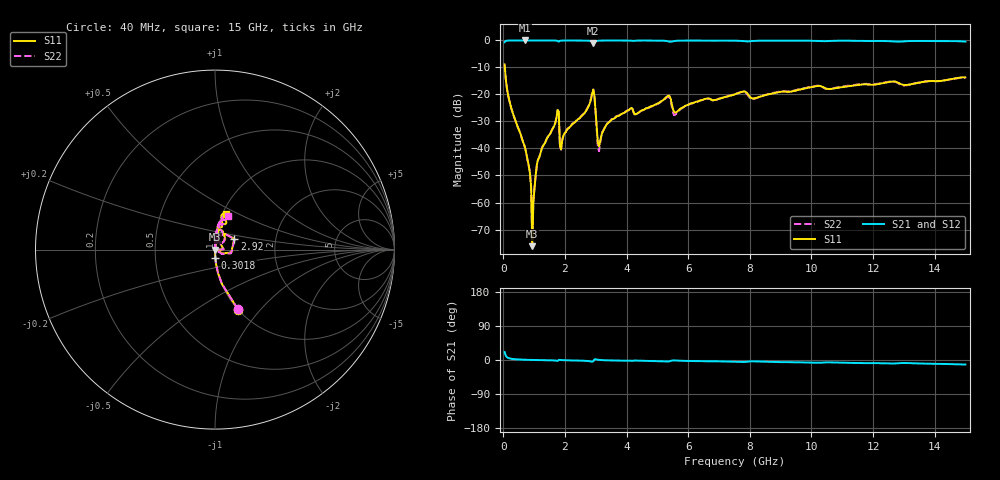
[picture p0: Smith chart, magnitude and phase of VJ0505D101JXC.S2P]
! VJ0505D101JXC
! MLCC placed on 25 mil thick microstrip substrate in series configuraton.
! DATE 06/29/2018  09:30
! CORRECTED  DATA
# GHz  S  MA  R  50.00
!  FREQ  S11M  S11A  S21M  S21A  S12M  S12A  S22M  S22A
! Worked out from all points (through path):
!   401 points, 40 MHz to 15 GHz, reference 50 ohm
!   highest |S21| = -0.02 dB at 713.2 MHz (marker M1); lowest = -1.0 dB at 2.92 GHz (marker M2)
!   group delay of S21, straight-line fit = 2.32 ps
!   lowest |S11| = -76.2 dB at 937.6 MHz (marker M3), VSWR 1.00, Z = 50 - j0.013 ohm
!   |S11| at or under -10 dB: 47.84 MHz to end of sweep
!   |S22| runs from -73.9 to -9.0 dB; largest |S21 - S12| = 0.0025
!   S11 on the Smith chart (normalised r, x): 40 MHz: 1.00, -0.77; 301.8 MHz: 1.00, -0.09; 2.92 GHz: 1.23, +0.15; 15 GHz: 1.04, +0.43
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0.04  0.3596 -68.9  0.9316 21.0  0.9329 21.0  0.3562 -69.0
0.3018  0.04595 -88.1  0.9967 2.7  0.9973 2.7  0.04554 -88.0
0.7132  0.009823 -88.4  0.9981 0.7  0.9983 0.7  0.009853 -89.1
0.9376  0.0001556 -56.8  0.9977 0.2  0.9983 0.3  0.0002026 -155.7
1.0124  0.001882 81.8  0.9977 0.0  0.9983 0.1  0.001957 98.7
1.0498  0.003275 83.6  0.9978 -0.0  0.9981 0.1  0.003158 88.3
1.162  0.006779 87.1  0.9976 -0.2  0.9979 -0.1  0.006868 91.2
1.723  0.03694 77.1  0.9906 -1.8  0.9903 -1.7  0.03705 77.9
1.91  0.01408 78.4  0.9937 -0.4  0.9951 -0.3  0.01431 81.0
2.5458  0.04019 85.5  0.9945 -1.8  0.995 -1.7  0.04103 85.3
2.9198  0.1232 29.7  0.8908 -3.1  0.8914 -3.0  0.1234 27.3
3.0694  0.01265 0.4  0.9861 0.7  0.9864 0.8  0.009905 -2.1
3.1442  0.01359 61.9  0.9919 -0.0  0.9924 0.0  0.01293 69.9
3.593  0.03573 85.1  0.9957 -1.3  0.9962 -1.3  0.03602 88.2
5.0516  0.07003 84.3  0.9921 -3.0  0.9924 -3.0  0.06866 84.7
5.3508  0.09494 65.9  0.9612 -4.0  0.9615 -3.9  0.09052 64.7
5.6126  0.04703 69.5  0.9836 -1.4  0.984 -1.4  0.04384 74.8
7.52  0.1011 81.9  0.9878 -4.7  0.9886 -4.7  0.1023 83.5
8.1184  0.08409 72.5  0.9777 -3.6  0.9783 -3.6  0.08218 76.9
10.0258  0.1385 81.9  0.9835 -7.0  0.9846 -7.0  0.1405 81.1
12.5316  0.1705 75.1  0.9677 -9.3  0.9682 -9.3  0.1722 75.9
15  0.2076 73.3  0.9512 -11.8  0.9519 -11.8  0.2014 69.3
